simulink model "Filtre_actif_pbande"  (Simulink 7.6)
settings: Solver=ode15s  StartTime=0.0  StopTime=0.02  RelTol=1e-3
InitFcn:
  | C=100e-9;
  | L=0.1;
  | R2=10e3;
  | R1=1e3;
StopFcn:
  | close all, clc
  | load passe_bande.mat
  | plot(x(1,:),x(2,:),x(1,:),x(3,:))
  | title('Entrée et sortie du filtre passe bande')
  | xlabel('temps')
  | grid
libraries: fl_lib x8, nesl_utility x3, elec_lib x2, simulink x1

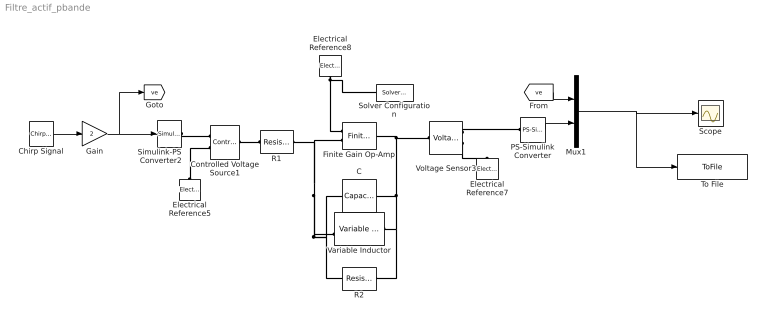
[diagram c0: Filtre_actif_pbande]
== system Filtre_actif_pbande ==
  C : fl_lib/Electrical/Electrical Elements/Capacitor  DialogController=NetworkEngine.DynNeDlgSource  SystemSampleTime=-1  c=C F  v0=0 V  r=0 Ohm  g=0 1/Ohm  i_Log=off  v_Log=off  vc_Log=off  LocalVarNames=|current|voltage|power  LocalVarDescs=|Capacitor current (A)|Voltage across capacitor (V)|Power (W)  LocalVarLogging=[0 0 0]
  Chirp Signal : simulink/Sources/Chirp Signal  SystemSampleTime=-1  f1=10  T=0.02  f2=5000
  Controlled Voltage Source1 : fl_lib/Electrical/Electrical Sources/Controlled Voltage Source  DialogController=NetworkEngine.DynNeDlgSource  SystemSampleTime=-1  i_Log=off  v_Log=off  LocalVarNames=|current|voltage|power  LocalVarDescs=|Current (A)|Voltage (V)|Power (W)  LocalVarLogging=[0 0 0]
  Electrical Reference5 : fl_lib/Electrical/Electrical Elements/Electrical Reference  DialogController=NetworkEngine.DynNeDlgSource  SystemSampleTime=-1  i_Log=off  LocalVarNames=|i  LocalVarDescs=|i  LocalVarLogging=[]
  Electrical Reference7 : fl_lib/Electrical/Electrical Elements/Electrical Reference  DialogController=NetworkEngine.DynNeDlgSource  SystemSampleTime=-1  i_Log=off  LocalVarNames=|i  LocalVarDescs=|i  LocalVarLogging=[]
  Electrical Reference8 : fl_lib/Electrical/Electrical Elements/Electrical Reference  DialogController=NetworkEngine.DynNeDlgSource  SystemSampleTime=-1  i_Log=off  LocalVarNames=|i  LocalVarDescs=|i  LocalVarLogging=[]
  Finite Gain Op-Amp : elec_lib/Integrated Circuits/Finite Gain Op-Amp  DialogController=NetworkEngine.DynNeDlgSource  SystemSampleTime=-1  A=1000  Rin=1e+06 Ohm  Rout=100 Ohm  Vmin=-15 V  Vmax=15 V  LocalVarNames=|power  LocalVarDescs=|Dissipated power (W)  LocalVarLogging=0
  Gain : Gain  Gain=2
  Mux1 : Mux  Inputs=2
  PS-Simulink Converter : nesl_utility/PS-Simulink Converter  DialogController=NetworkEngine.DynNeUtilDlgSource  SystemSampleTime=-1  PhysicalDomain=network_engine_domain  LeftPortType=input  RightPortType=output  SubClassName=ps_output  Unit=1  AffineConversion=off
  R1 : fl_lib/Electrical/Electrical Elements/Resistor  DialogController=NetworkEngine.DynNeDlgSource  SystemSampleTime=-1  R=R1 Ohm  i_Log=off  v_Log=off  LocalVarNames=|current|voltage|power  LocalVarDescs=|Resistor current (A)|Voltage across resistor (V)|Power (W)  LocalVarLogging=[0 0 0]
  R2 : fl_lib/Electrical/Electrical Elements/Resistor  DialogController=NetworkEngine.DynNeDlgSource  SystemSampleTime=-1  R=R2 Ohm  i_Log=off  v_Log=off  LocalVarNames=|current|voltage|power  LocalVarDescs=|Resistor current (A)|Voltage across resistor (V)|Power (W)  LocalVarLogging=[0 0 0]
  Scope : Scope
  Simulink-PS Converter2 : nesl_utility/Simulink-PS Converter  DialogController=NetworkEngine.DynNeUtilDlgSource  SystemSampleTime=-1  PhysicalDomain=network_engine_domain  LeftPortType=input  RightPortType=output  SubClassName=ps_input  Unit=1  AffineConversion=off  InputFilterTimeConstant=.001  UdotUserProvided=0
  Solver Configuration : nesl_utility/Solver Configuration  DialogController=NetworkEngine.DynNeUtilDlgSource  SystemSampleTime=-1  PhysicalDomain=network_engine_domain  LeftPortType=input  RightPortType=generic  SubClassName=solver  Accelerate=off  Profile=off  ResidualTolerance=1e-40  MaxNonlinIter=12  MaxModeIter=2  DoFixedCost=off  UseLocalSampling=off  DoDC=on  LinearAlgebra=Full  LocalSolverSampleTime=.001  LocalSolverChoice=NE_BACKWARD_EULER_ADVANCER  UseLocalSolver=off
  To File : ToFile  Filename=passe_bande  MatrixName=x
  Variable Inductor : elec_lib/Passive Devices/Variable Inductor  DialogController=NetworkEngine.DynNeDlgSource  SystemSampleTime=-1  prm=1  Lmin=L H  g=0 1/Ohm  i0=0 A  phi0=0 Wb  LocalVarLogging=[]
  Voltage Sensor3 : fl_lib/Electrical/Electrical Sensors/Voltage Sensor  DialogController=NetworkEngine.DynNeDlgSource  SystemSampleTime=-1  i1_Log=off  v1_Log=off  LocalVarNames=|i1|v1  LocalVarDescs=|i1|v1  LocalVarLogging=[]
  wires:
  Chirp Signal/1 -> Gain/1
  PS-Simulink Converter/1 -> Mux1/2
  Mux1/1 -> To File/1, Scope/1
  [ve] -> Mux1/1
  Gain/1 -> Simulink-PS Converter2/1, [ve]
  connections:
  Controlled Voltage Source1/LConn1 -- R1/RConn1
  Simulink-PS Converter2/RConn1 -- Controlled Voltage Source1/RConn1
  Electrical Reference5/LConn1 -- Controlled Voltage Source1/RConn2
  Voltage Sensor3/RConn2 -- Electrical Reference7/LConn1
  Voltage Sensor3/RConn1 -- PS-Simulink Converter/LConn1
  Variable Inductor/RConn1 -- C/RConn1 -- Finite Gain Op-Amp/RConn1 -- Voltage Sensor3/LConn1 -- R2/LConn1
  Electrical Reference8/LConn1 -- Finite Gain Op-Amp/LConn1 -- Solver Configuration/RConn1
  Finite Gain Op-Amp/LConn2 -- R1/LConn1 -- C/LConn1 -- Variable Inductor/LConn2 -- R2/RConn1
